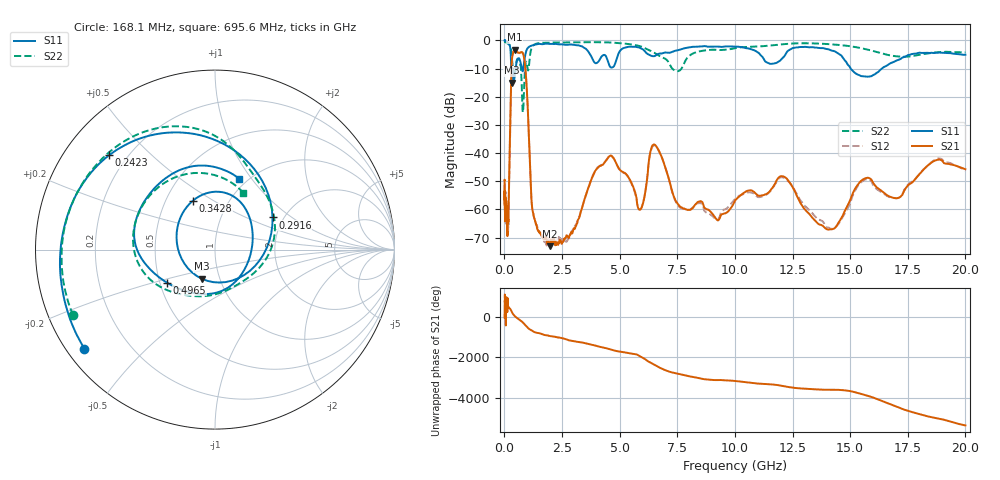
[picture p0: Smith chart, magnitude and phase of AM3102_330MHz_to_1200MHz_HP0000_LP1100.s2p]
! Date/Time: Tue, Sep 11, 2018 5:09 PM
! Network Analyzer: Agilent Technologies E8362B Rev: A.07.50.63
! Sweep from 0.010 to 20.000 GHz, 1601 Points, Sweep Type: LOG
! Power Supply: 4.950 V, 0.001 A
# Hz S DB R 50
!freq MagS11 AngS11 MagS21 AngS21 MagS12 AngS12 MagS22 AngS22
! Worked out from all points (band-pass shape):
!   1601 points, 10 MHz to 20 GHz, reference 50 ohm
!   highest |S21| = -3.29 dB at 455.8 MHz (marker M1); lowest = -73.0 dB at 1.96 GHz (marker M2)
!   |S21| within 3 dB of the highest: 333.7 MHz to 856.4 MHz (522.6 MHz wide, 87.8 % of centre)
!   lowest |S11| = -15.0 dB at 314.7 MHz (marker M3), VSWR 1.43, Z = 41.1 - j13.8 ohm
!   |S11| at or under -10 dB: 363.8 MHz to 493.7 MHz (129.9 MHz wide, 30.3 % of centre); 757.2 MHz to 822.7 MHz (65.53 MHz wide, 8.3 % of centre); 15.03 GHz to 16.37 GHz (1.348 GHz wide, 8.59 % of centre)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
!   |S22| runs from -25.5 to -0.3 dB; largest |S21 - S12| = 0.012
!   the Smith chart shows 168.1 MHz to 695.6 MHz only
!   S11 on the Smith chart (normalised r, x): 168.1 MHz: 0.05, -0.34; 242.3 MHz: 0.13, +0.38; 291.6 MHz: 1.75, +0.72; 342.8 MHz: 0.68, +0.41; 496.5 MHz: 0.55, -0.22; 695.6 MHz: 0.91, +0.87
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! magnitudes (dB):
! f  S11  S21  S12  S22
! 10 MHz  0.0  -49.5  -54.0  -0.3
! 35.55 MHz  0.0  -58.4  -59.9  -0.5
! 126.4 MHz  -0.4  -67.1  -64.3  -1.0
! 168.1 MHz  -0.8  -64.0  -65.1  -1.2
! 242.3 MHz  -2.0  -34.2  -34.3  -1.8
! 291.6 MHz  -8.7  -13.8  -13.9  -3.5
! 314.7 MHz  -15.0  -8.3  -8.3  -5.6
! 342.8 MHz  -10.5  -5.8  -5.8  -7.6
! 447.2 MHz  -12.7  -3.3  -3.3  -11.8
! 455.8 MHz  -12.3  -3.3  -3.3  -11.5
! 496.5 MHz  -9.8  -3.4  -3.6  -9.3
! 695.6 MHz  -7.6  -4.3  -4.3  -9.0
! 806 MHz  -10.7  -4.6  -4.7  -25.5
! 1.201 GHz  -1.8  -59.1  -59.2  -2.3
! 1.59 GHz  -1.3  -68.9  -68.7  -0.9
! 1.96 GHz  -1.2  -73.0  -70.3  -0.8
! 4.543 GHz  -8.6  -41.2  -41.1  -0.7
! 5.652 GHz  -2.2  -53.4  -53.7  -1.6
! 6.58 GHz  -5.2  -37.5  -37.6  -4.8
! 7.734 GHz  -2.9  -59.5  -59.7  -9.3
! 14.01 GHz  -3.1  -67.1  -66.4  -1.3
! 20 GHz  -5.1  -45.7  -46.2  -4.2
